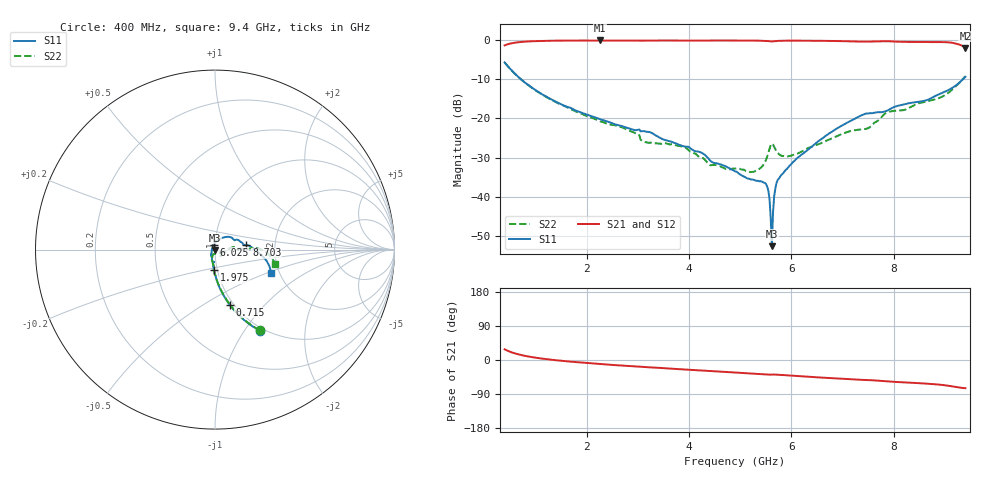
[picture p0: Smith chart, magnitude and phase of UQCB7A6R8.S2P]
!  Part Number  UQCB7A6R8	Mounting Orientation: Vertical
!  Description: RF capacitors
!  Application: Coupling, Bypass, Tuning, DC Block
!  Filters, Matching
# GHZ S DB R 50
! Freq  |S11|  S11 Ph  |S21|  S21 Ph  |S12|  S12 Ph  |S22|  S22 Ph
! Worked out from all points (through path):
!   401 points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, 400 MHz to 9.4 GHz, reference 50 ohm
!   highest |S21| = -0.16 dB at 2.268 GHz (marker M1); lowest = -2.0 dB at 9.4 GHz (marker M2)
!   group delay of S21, straight-line fit = 24.9 ps
!   lowest |S11| = -52.5 dB at 5.62 GHz (marker M3), VSWR 1.00, Z = 50.1 - j0.227 ohm
!   |S11| at or under -10 dB: 715.9 MHz to 9.354 GHz (8.638 GHz wide, 172 % of centre)
!   |S22| runs from -33.6 to -5.8 dB; largest |S21 - S12| = 0.0045
!   S11 on the Smith chart (normalised r, x): 400 MHz: 0.96, -1.18; 715 MHz: 0.96, -0.65; 1.975 GHz: 0.96, -0.22; 6.025 GHz: 0.98, +0.05; 8.703 GHz: 1.42, +0.07; 9.4 GHz: 1.81, -0.53
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0.4  -5.74 -61.0  -1.42 28.2  -1.43 28.2  -5.76 -60.9
0.715  -9.99 -75.2  -0.55 13.4  -0.55 13.3  -10.01 -74.9
1.908  -18.57 -92.2  -0.17 -6.9  -0.18 -6.9  -18.85 -93.1
1.975  -18.85 -92.8  -0.17 -7.6  -0.17 -7.6  -19.21 -94.0
2.268  -20.21 -95.3  -0.16 -10.7  -0.19 -10.7  -20.72 -95.1
3.415  -24.79 -107.7  -0.17 -20.7  -0.20 -20.6  -26.40 -99.3
3.888  -27.06 -114.7  -0.19 -24.8  -0.21 -24.8  -27.16 -108.7
4.405  -30.59 -133.8  -0.19 -28.8  -0.21 -28.7  -31.80 -106.8
4.9  -33.45 -151.3  -0.17 -33.0  -0.20 -33.0  -32.73 -81.1
5.26  -35.57 172.7  -0.20 -36.1  -0.22 -36.0  -33.58 -57.9
5.485  -36.39 120.7  -0.25 -38.1  -0.27 -38.0  -31.11 -31.8
5.53  -37.40 100.3  -0.29 -38.5  -0.31 -38.5  -29.65 -27.6
5.575  -40.62 68.3  -0.36 -38.8  -0.38 -38.8  -27.64 -29.7
5.62  -52.49 -73.0  -0.41 -38.5  -0.43 -38.4  -26.36 -42.9
5.733  -35.67 153.0  -0.27 -38.9  -0.29 -38.8  -28.80 -55.3
6.025  -31.21 107.3  -0.20 -41.5  -0.21 -41.5  -29.37 -36.9
6.408  -27.12 81.6  -0.24 -44.9  -0.26 -44.8  -27.15 -22.9
7.33  -19.46 41.7  -0.44 -52.1  -0.45 -52.0  -22.82 -7.2
7.915  -17.71 25.2  -0.37 -56.7  -0.38 -56.6  -18.28 2.1
8.703  -15.04 8.1  -0.57 -63.0  -0.58 -62.9  -15.46 -0.5
9.13  -12.33 -3.7  -0.73 -69.4  -0.74 -69.3  -12.80 2.1
9.4  -9.41 -22.5  -2.04 -74.4  -2.05 -74.3  -9.25 -13.7
